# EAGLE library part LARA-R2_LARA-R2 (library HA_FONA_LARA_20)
LARA-R2 series: Size-optimized LTE Cat 1 modules in single and multi-mode configurations
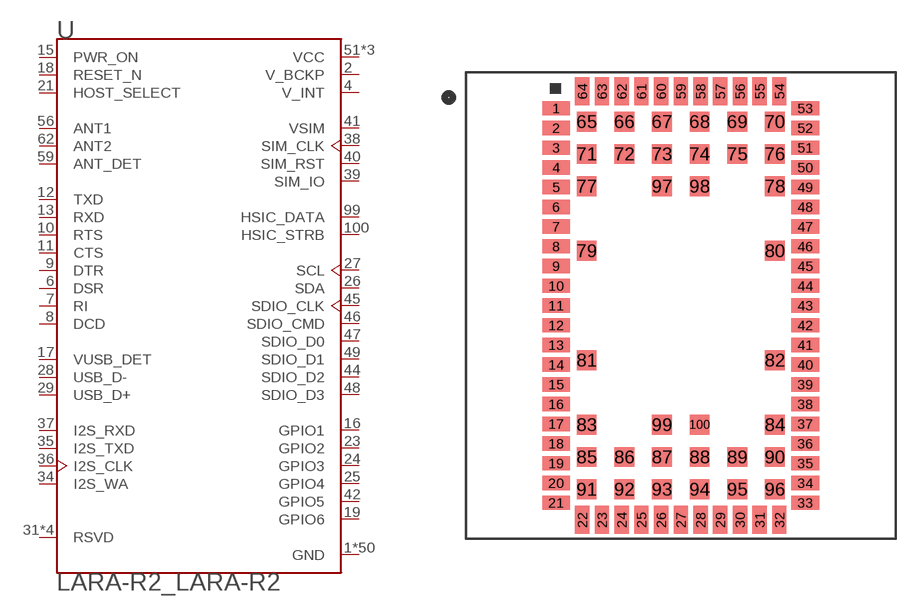
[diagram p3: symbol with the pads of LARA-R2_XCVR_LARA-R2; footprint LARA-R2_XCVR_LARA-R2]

Designator prefix U

## LARA-R2_LARA-R2 (AVAILABILITY: Unavailable; DESCRIPTION: Cellular 4G LTE CAT-1 (Verizon) Transceiver Module 900MHz, 1.8GHz Antenna Not Included, Castellation Surface Mount; MF: U-Blox America; MP: LARA-R2; PACKAGE: SMD-100 U-Blox America; PRICE: None)  [LARA-R2_XCVR_LARA-R2]
1  GND  pwr
2  V_BCKP  pwr
3  GND  pwr
4  V_INT  pwr
5  GND  pwr
6  DSR  out
7  RI  out
8  DCD  out
9  DTR  in
10  RTS  in
11  CTS  out
12  TXD  in
13  RXD  out
14  GND  pwr
15  PWR_ON  in
16  GPIO1
17  VUSB_DET  in
18  RESET_N  in
19  GPIO6  out
20  GND  pwr
21  HOST_SELECT
22  GND  pwr
23  GPIO2
24  GPIO3
25  GPIO4
26  SDA
27  SCL  out
28  USB_D-
29  USB_D+
30  GND  pwr
31  RSVD  pas
32  GND  pwr
33  RSVD  pas
34  I2S_WA
35  I2S_TXD
36  I2S_CLK
37  I2S_RXD
38  SIM_CLK  out
39  SIM_IO
40  SIM_RST  out
41  VSIM  out
42  GPIO5
43  GND  pwr
44  SDIO_D2
45  SDIO_CLK  out
46  SDIO_CMD
47  SDIO_D0
48  SDIO_D3
49  SDIO_D1
50  GND  pwr
51  VCC  pwr
52  VCC  pwr
53  VCC  pwr
54  GND  pwr
55  GND  pwr
56  ANT1
57  GND  pwr
58  GND  pwr
59  ANT_DET  in
60  GND  pwr
61  GND  pwr
62  ANT2  in
63  GND  pwr
64  GND  pwr
65  GND  pwr
66  GND  pwr
67  GND  pwr
68  GND  pwr
69  GND  pwr
70  GND  pwr
71  GND  pwr
72  GND  pwr
73  GND  pwr
74  GND  pwr
75  GND  pwr
76  GND  pwr
77  GND  pwr
78  GND  pwr
79  GND  pwr
80  GND  pwr
81  GND  pwr
82  GND  pwr
83  GND  pwr
84  GND  pwr
85  GND  pwr
86  GND  pwr
87  GND  pwr
88  GND  pwr
89  GND  pwr
90  GND  pwr
91  GND  pwr
92  GND  pwr
93  GND  pwr
94  GND  pwr
95  GND  pwr
96  GND  pwr
97  RSVD  pas
98  RSVD  pas
99  HSIC_DATA
100  HSIC_STRB

## Footprint LARA-R2_XCVR_LARA-R2 (pad centres in mm)
smd 1.55 x 0.8: 1 -6.95,11; 2 -6.95,9.9; 3 -6.95,8.8; 4 -6.95,7.7; 5 -6.95,6.6; 6 -6.95,5.5; 7 -6.95,4.4; 8 -6.95,3.3; 9 -6.95,2.2; 10 -6.95,1.1; 11 -6.95,0; 12 -6.95,-1.1; 13 -6.95,-2.2; 14 -6.95,-3.3; 15 -6.95,-4.4; 16 -6.95,-5.5; 17 -6.95,-6.6; 18 -6.95,-7.7; 19 -6.95,-8.8; 20 -6.95,-9.9; 21 -6.95,-11; 33 6.95,-11; 34 6.95,-9.9; 35 6.95,-8.8; 36 6.95,-7.7; 37 6.95,-6.6; 38 6.95,-5.5; 39 6.95,-4.4; 40 6.95,-3.3; 41 6.95,-2.2; 42 6.95,-1.1; 43 6.95,0; 44 6.95,1.1; 45 6.95,2.2; 46 6.95,3.3; 47 6.95,4.4; 48 6.95,5.5; 49 6.95,6.6; 50 6.95,7.7; 51 6.95,8.8; 52 6.95,9.9; 53 6.95,11
smd 0.8 x 1.55: 22 -5.5,-11.95; 23 -4.4,-11.95; 24 -3.3,-11.95; 25 -2.2,-11.95; 26 -1.1,-11.95; 27 0,-11.95; 28 1.1,-11.95; 29 2.2,-11.95; 30 3.3,-11.95; 31 4.4,-11.95; 32 5.5,-11.95; 54 5.5,11.95; 55 4.4,11.95; 56 3.3,11.95; 57 2.2,11.95; 58 1.1,11.95; 59 0,11.95; 60 -1.1,11.95; 61 -2.2,11.95; 62 -3.3,11.95; 63 -4.4,11.95; 64 -5.5,11.95
smd 1.1 x 1.1: 65 -5.25,10.25; 66 -3.15,10.25; 67 -1.05,10.25; 68 1.05,10.25; 69 3.15,10.25; 70 5.25,10.25; 71 -5.25,8.45; 72 -3.15,8.45; 73 -1.05,8.45; 74 1.05,8.45; 75 3.15,8.45; 76 5.25,8.45; 77 -5.25,6.65; 78 5.25,6.65; 79 -5.25,3.05; 80 5.25,3.05; 81 -5.25,-3.05; 82 5.25,-3.05; 83 -5.25,-6.65; 84 5.25,-6.65; 85 -5.25,-8.45; 86 -3.15,-8.45; 87 -1.05,-8.45; 88 1.05,-8.45; 89 3.15,-8.45; 90 5.25,-8.45; 91 -5.25,-10.25; 92 -3.15,-10.25; 93 -1.05,-10.25; 94 1.05,-10.25; 95 3.15,-10.25; 96 5.25,-10.25; 97 -1.05,6.65; 98 1.05,6.65; 99 -1.05,-6.65; 100 1.05,-6.65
